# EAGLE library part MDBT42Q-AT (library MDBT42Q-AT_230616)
Raytac Corporation Part Number: (nRF52810) MDBT42Q-AT / MDBT42Q-PAT (nRF52811) MDBT42Q-ATL / MDBT42Q-PATL Bluetooth Low Energy Module based on Noridc nRF52810 / nRF52811 Size: 16x10mm Source: Raytac datasheet
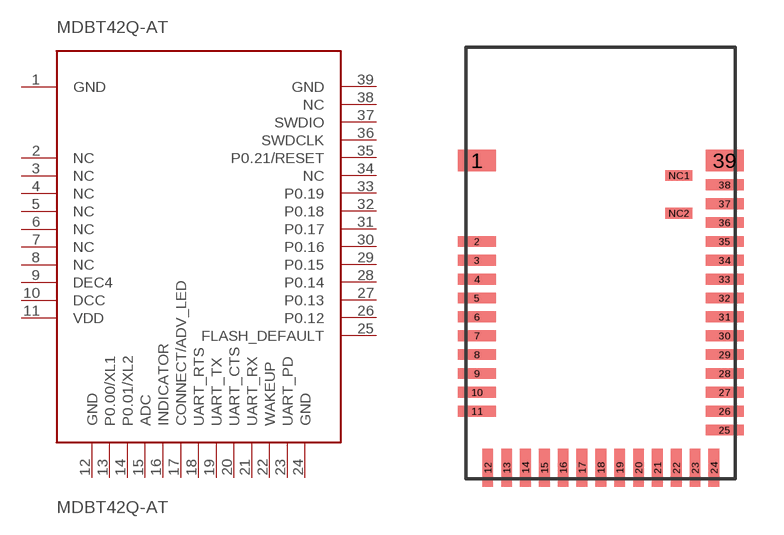
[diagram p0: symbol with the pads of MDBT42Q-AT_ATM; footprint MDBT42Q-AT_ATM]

Designator prefix MDBT42Q-AT

## MDBT42Q-AT  [MDBT42Q-AT_ATM]
1  GND
2  NC
3  NC
4  NC
5  NC
6  NC
7  NC
8  NC
9  DEC4
10  DCC
11  VDD
12  GND
13  P0.00/XL1
14  P0.01/XL2
15  ADC
16  INDICATOR
17  CONNECT/ADV_LED
18  UART_RTS
19  UART_TX
20  UART_CTS
21  UART_RX
22  WAKEUP
23  UART_PD
24  GND
25  FLASH_DEFAULT
26  P0.12
27  P0.13
28  P0.14
29  P0.15
30  P0.16
31  P0.17
32  P0.18
33  P0.19
34  NC
35  P0.21/RESET
36  SWDCLK
37  SWDIO
38  NC
39  GND

## Footprint MDBT42Q-AT_ATM (pad centres in mm)
Raytac Corporation Part Number: (nRF52832) MDBT42Q-ATM / MDBT42Q-PATM (nRF52810) MDBT42Q-AT / MDBT42Q-PAT (nRF52811) MDBT42Q-ATL / MDBT42Q-PATL Bluetooth Low Energy Module based on Noridc nRF52832 /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
smd 1.4 x 0.8: 1 -4.6,3.8; 39 4.6,3.8
smd 1.4 x 0.4: 2 -4.6,0.8; 3 -4.6,0.1; 4 -4.6,-0.6; 5 -4.6,-1.3; 6 -4.6,-2; 7 -4.6,-2.7; 8 -4.6,-3.4; 9 -4.6,-4.1; 10 -4.6,-4.8; 11 -4.6,-5.5; 25 4.6,-6.2; 26 4.6,-5.5; 27 4.6,-4.8; 28 4.6,-4.1; 29 4.6,-3.4; 30 4.6,-2.7; 31 4.6,-2; 32 4.6,-1.3; 33 4.6,-0.6; 34 4.6,0.1; 35 4.6,0.8; 36 4.6,1.5; 37 4.6,2.2; 38 4.6,2.9
smd 0.4 x 1.4: 12 -4.2,-7.6; 13 -3.5,-7.6; 14 -2.8,-7.6; 15 -2.1,-7.6; 16 -1.4,-7.6; 17 -0.7,-7.6; 18 0,-7.6; 19 0.7,-7.6; 20 1.4,-7.6; 21 2.1,-7.6; 22 2.8,-7.6; 23 3.5,-7.6; 24 4.2,-7.6
smd 1 x 0.4: NC1 2.9,3.25; NC2 2.9,1.85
